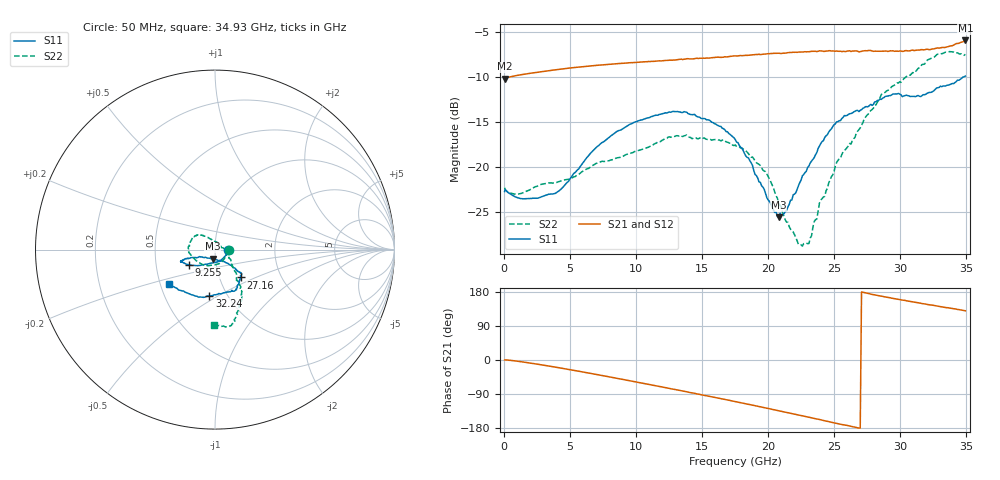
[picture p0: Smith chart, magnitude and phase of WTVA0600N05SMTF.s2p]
! 50 ohm 2-Port S-parameters measured by Modelithics Inc support@modelithics.com  Tampa, FL USA 813-866-6335 (February 2024)
! Smiths Interconnect,  6dB P/N: WTVA0600N05SMTF, Temperature: -50 C
! Board: 10 mil Rogers 4350B, Mounting Pad Dimensions: Length: 15 mils, Width: 25 mils, Gap: 40 mils.
# Hz S RI R 50
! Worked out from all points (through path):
!   352 points, 50 MHz to 34.93 GHz, reference 50 ohm
!   highest |S21| = -5.96 dB at 34.93 GHz (marker M1); lowest = -10.2 dB at 50 MHz (marker M2)
!   group delay of S21, straight-line fit = 19.2 ps
!   lowest |S11| = -25.6 dB at 20.8 GHz (marker M3), VSWR 1.11, Z = 48.5 - j4.95 ohm
!   |S11| at or under -10 dB: start of sweep to 34.8 GHz
!   |S22| runs from -28.8 to -7.2 dB; largest |S21 - S12| = 0.003
!   S11 on the Smith chart (normalised r, x): 50 MHz: 1.16, -0.01; 9.255 GHz: 0.74, -0.13; 27.16 GHz: 1.26, -0.41; 32.24 GHz: 0.83, -0.45; 34.93 GHz: 0.56, -0.23
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5e7  0.0728 -0.00293  0.309 0.00115  0.3089 0.00114  0.0765 -0.00281
9.96e8  0.0589 -0.0329  0.3214 -0.0174  0.3213 -0.0174  0.0601 -0.0366
3.8815e9  -0.000224 -0.0712  0.3273 -0.111  0.3271 -0.1111  0.016 -0.0799
5.8715e9  -0.0601 -0.0832  0.3081 -0.1851  0.3079 -0.1851  -0.029 -0.0889
9.2545e9  -0.1442 -0.0848  0.2272 -0.3012  0.227 -0.3011  -0.094 -0.0697
1.1742e10  -0.1823 -0.0699  0.1347 -0.3637  0.1342 -0.3637  -0.135 -0.0292
1.44285e10  -0.1853 -0.0627  0.0147 -0.3986  0.0141 -0.3984  -0.1431 0.0256
1.7513e10  -0.1342 -0.0448  -0.1401 -0.3889  -0.1403 -0.3887  -0.1061 0.0787
1.98015e10  -0.0568 -0.0426  -0.2517 -0.3397  -0.2512 -0.3399  -0.0566 0.0751
2.07965e10  -0.0128 -0.0509  -0.298 -0.3065  -0.2981 -0.3062  -0.0238 0.0585
2.13935e10  0.00791 -0.0567  -0.3193 -0.2864  -0.3194 -0.2861  -0.00822 0.0486
2.2289e10  0.0444 -0.0646  -0.3553 -0.249  -0.3556 -0.2484  0.0189 0.032
2.3085e10  0.067 -0.0758  -0.381 -0.2112  -0.3809 -0.2111  0.0359 0.011
2.33835e10  0.0757 -0.0797  -0.3917 -0.1967  -0.3916 -0.1964  0.0451 0.00994
2.3682e10  0.0838 -0.0859  -0.3979 -0.1791  -0.3977 -0.1791  0.0512 -0.00353
2.3881e10  0.0935 -0.0909  -0.406 -0.1717  -0.4058 -0.1716  0.0621 -0.0105
2.4279e10  0.1046 -0.101  -0.4122 -0.1473  -0.4121 -0.147  0.0617 -0.0297
2.51745e10  0.1291 -0.1221  -0.4288 -0.0971  -0.4286 -0.097  0.0883 -0.0576
2.71645e10  0.1432 -0.1553  -0.4398 0.00904  -0.4397 0.00921  0.1179 -0.1305
2.91545e10  0.1184 -0.2186  -0.4232 0.1152  -0.4229 0.1156  0.1428 -0.2275
3.2239e10  -0.0312 -0.2569  -0.3688 0.2532  -0.3694 0.2522  0.1139 -0.3802
3.49255e10  -0.257 -0.1896  -0.3229 0.3862  -0.3211 0.3873  -0.00827 -0.4213
